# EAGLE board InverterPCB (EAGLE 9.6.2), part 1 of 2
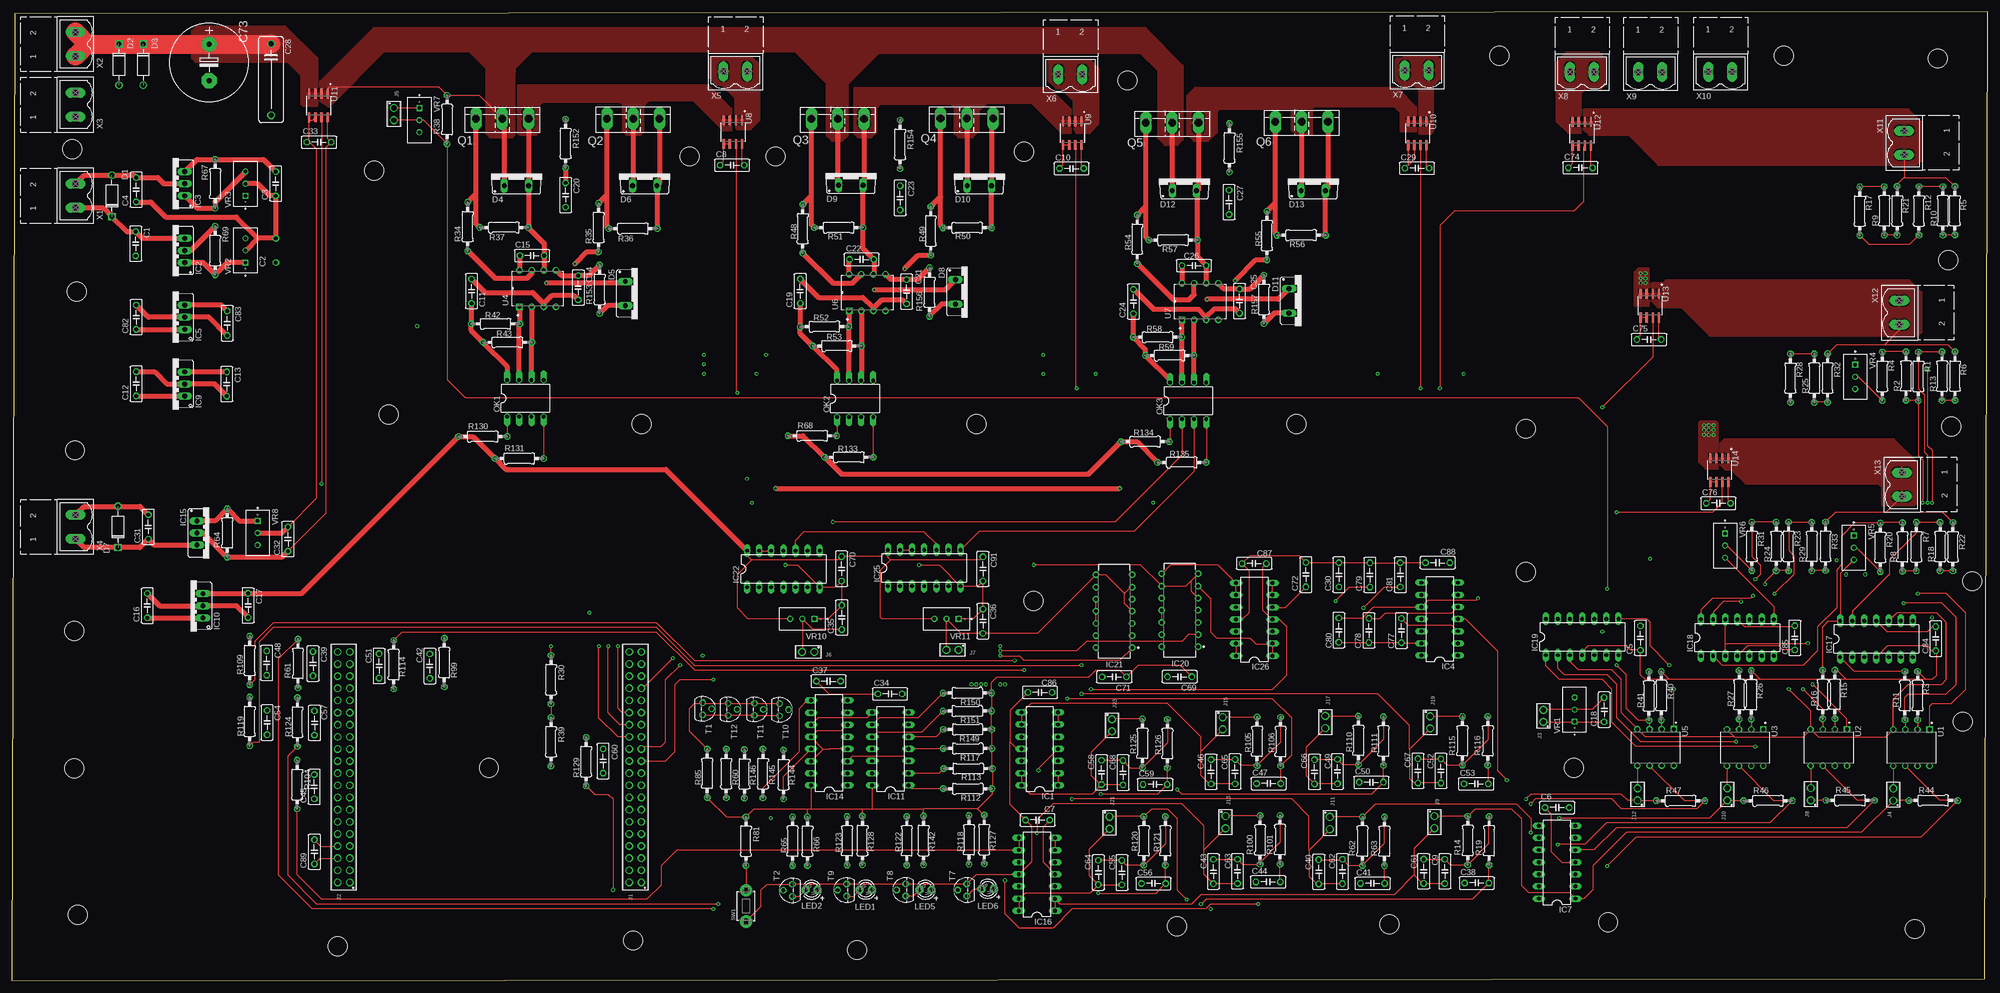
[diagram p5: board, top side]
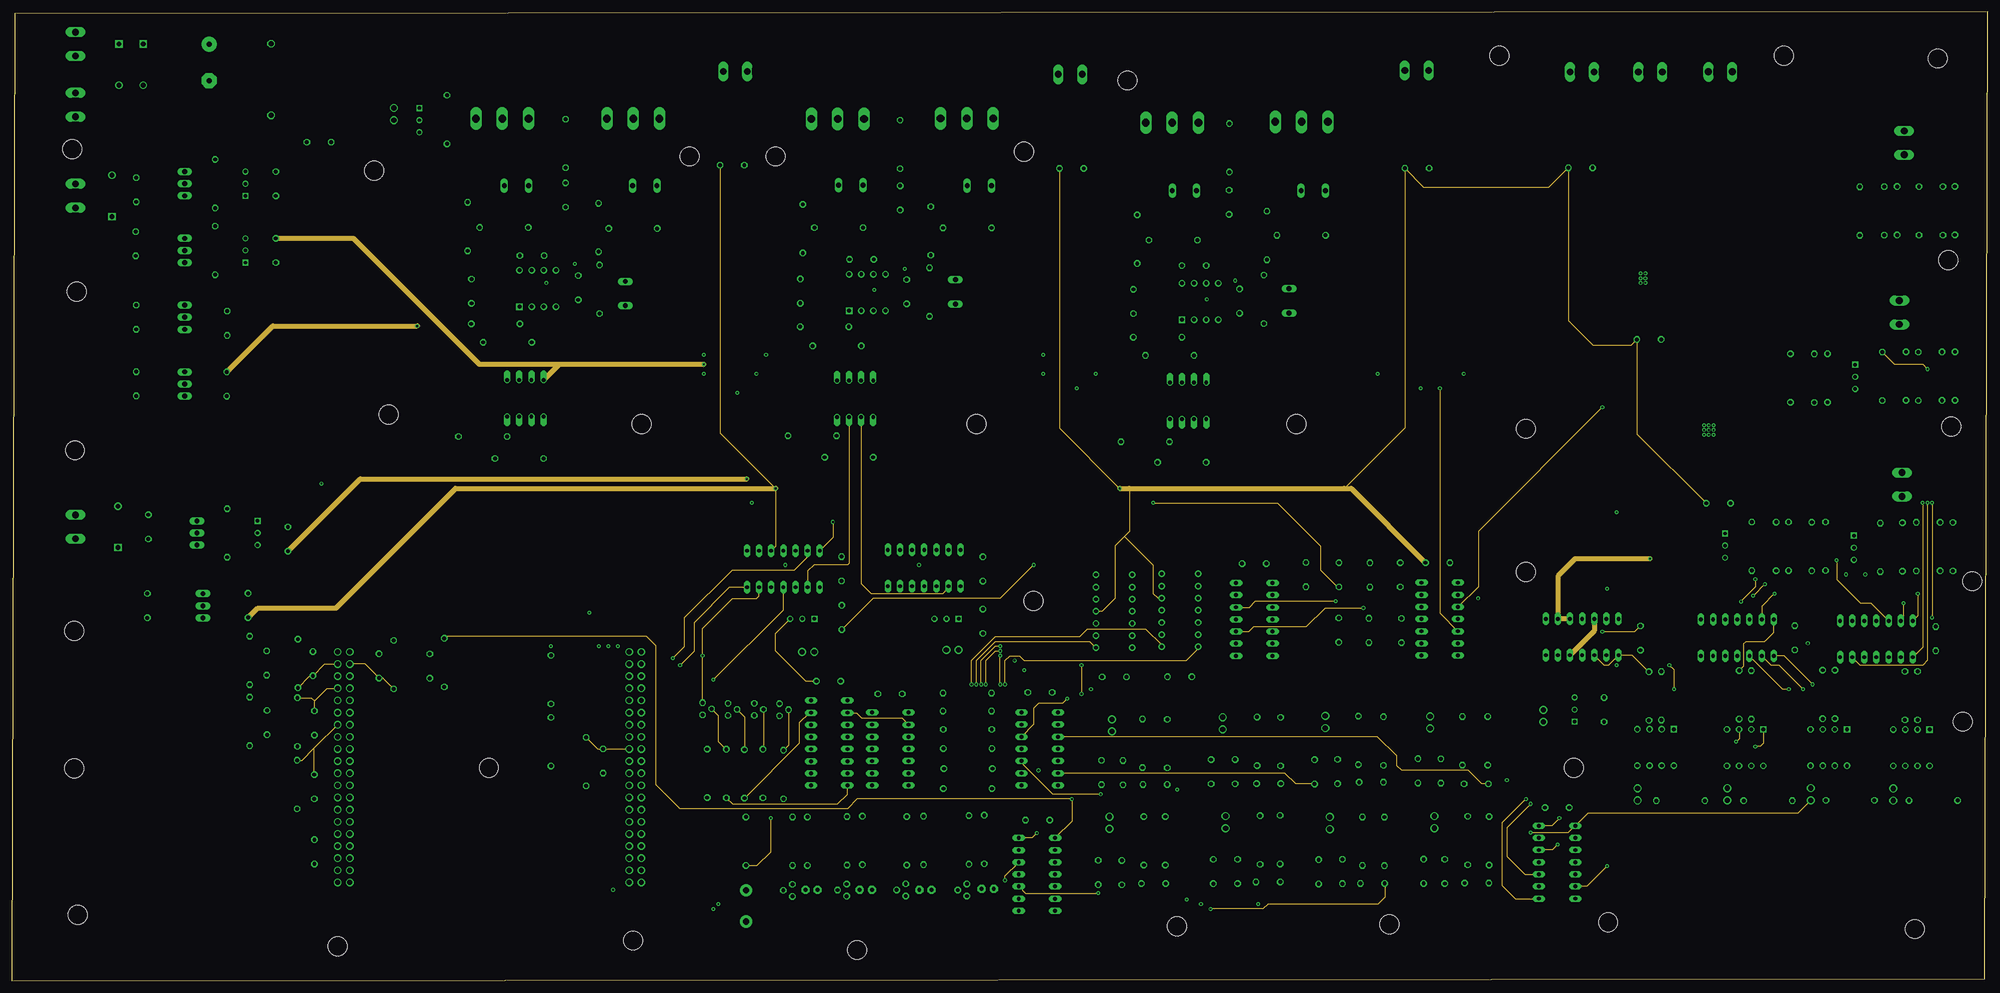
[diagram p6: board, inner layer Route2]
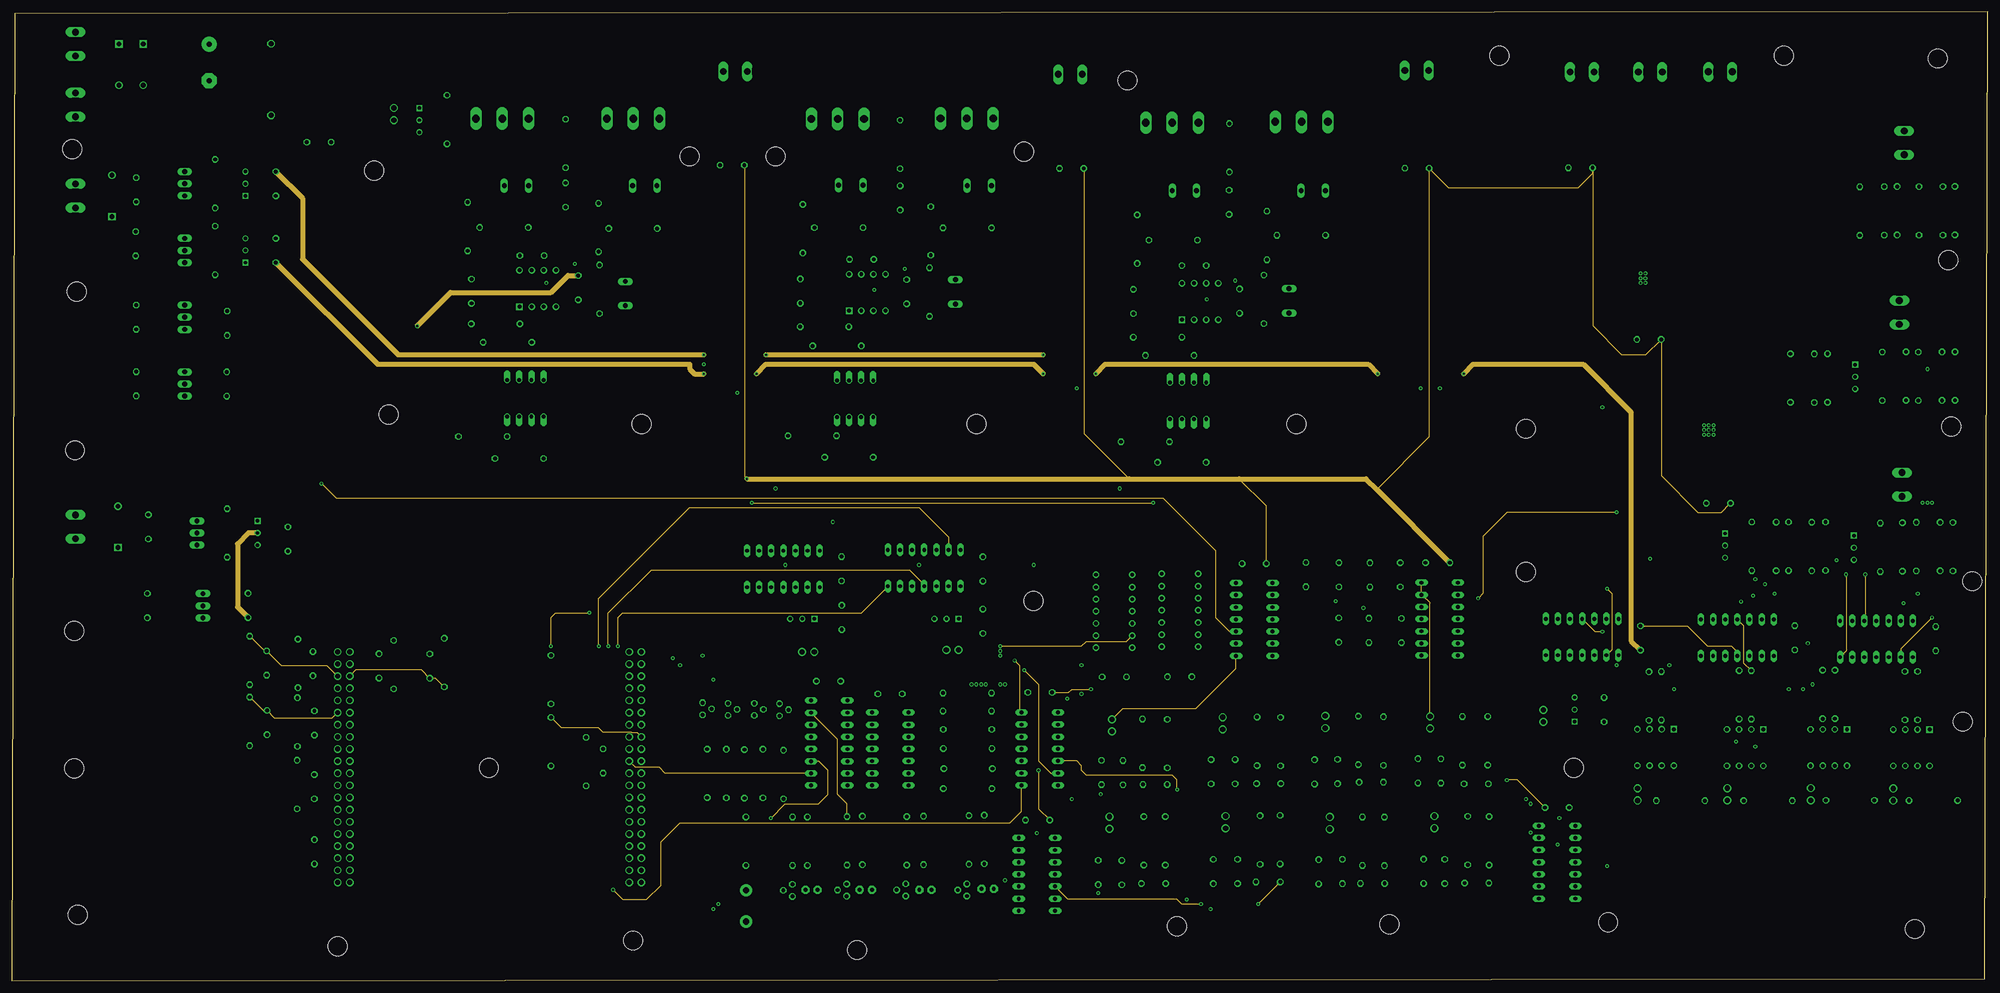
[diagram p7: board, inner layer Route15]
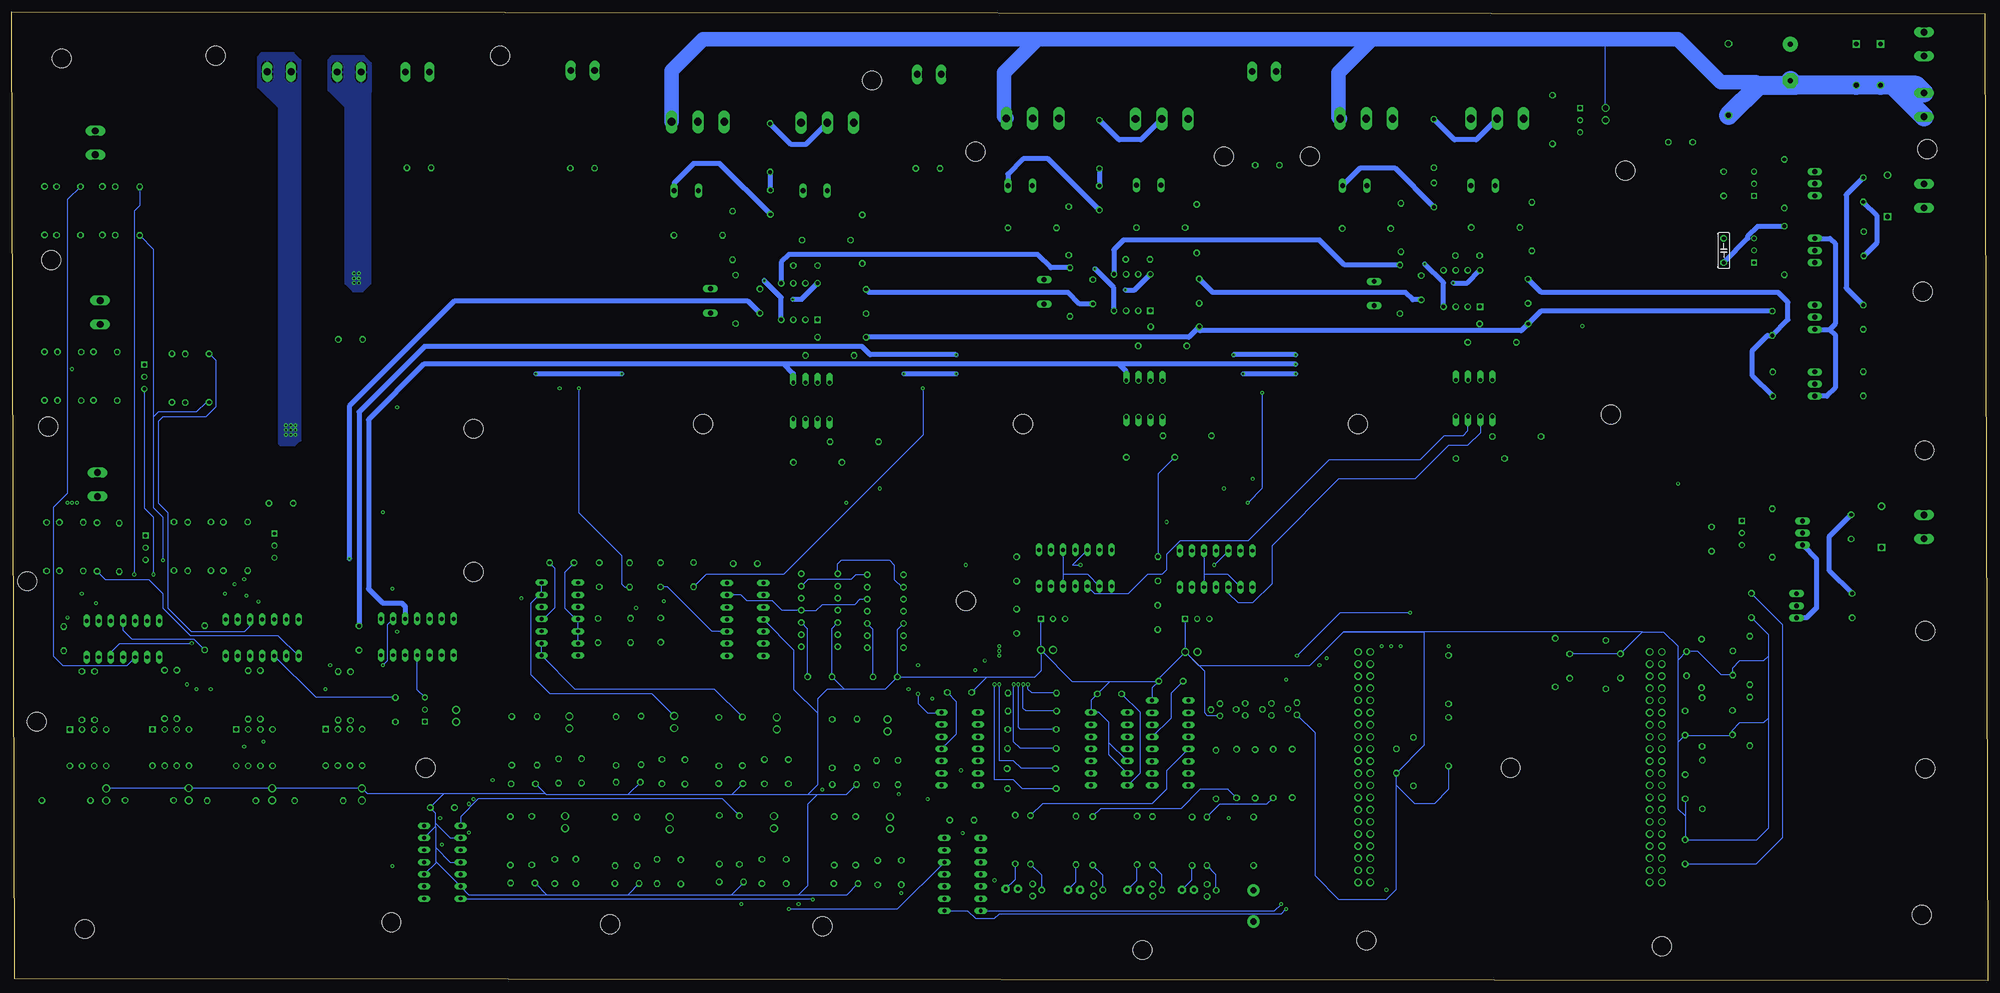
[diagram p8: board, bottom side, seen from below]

Size 413.38 x 202.75 mm. Coordinates in mm from the lower left corner, seen from the top.
Outline: 0,0 412.78,0.4 413.38,202.75 0.6,202.35 0,0
Copper layers (1+2*15+16): Top 0.07mm / dielectric 0.2mm / Route2 0.017mm / dielectric 1.465mm / Route15 0.017mm / dielectric 0.2mm / Bottom 0.07mm
Design rules "default *": minimum track width 6mil, minimum drill 0.35mm, track to track 6mil, track to pad 6mil, pad to pad 6mil, via to via 6mil, smd to smd 6mil, copper to edge 40mil, drill to drill 6mil, minimum pad ring 10mil, minimum via ring 8mil, stop-mask expansion 4mil, vias tented up to drill 0mil, thermal gap 10mil
Net classes: 1 High_gnd: clearance 1 mm
Holes 4 mm at 12.59,174.01 13.59,144.21 13.19,111.01 12.99,73.21 12.99,44.41 13.79,13.81 68.19,7.21 129.99,8.41 176.79,6.41 243.79,11.41 288.19,11.81 333.99,12.21 398.19,10.81 408.19,54.21 370.79,193.61 402.99,193.01 410.19,83.61 405.79,116.01 405.19,150.81 311.19,193.61 233.39,188.41 211.79,173.51 159.79,172.51 141.79,172.51 75.79,169.51 99.79,44.51 78.79,118.51 131.79,116.51 201.79,116.51 268.79,116.51 316.79,115.51 316.79,85.51 326.79,44.51 213.79,79.51

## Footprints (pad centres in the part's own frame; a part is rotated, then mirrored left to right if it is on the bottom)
C050-025X075 = drill 0.813 octagon: 1 -2.54,0; 2 2.54,0
C150-054X183 = drill 1.016 octagon: 1 -7.493,0; 2 7.493,0
E7,5-16 = drill 1.016 pad 3.15: + -3.81,0 | drill 1.016 pad 3.15 octagon: - 3.81,0
DO-41 = drill 1: A 4.325,0 | drill 1 square: C -4.325,0
TO220ACS = drill 1.016 long: A 2.54,-2.54; C -2.54,-2.54
DIL14 = drill 0.813 long: 1 -7.62,-3.81; 2 -5.08,-3.81; 3 -2.54,-3.81; 4 0,-3.81; 5 2.54,-3.81; 6 5.08,-3.81; 7 7.62,-3.81; 8 7.62,3.81; 9 5.08,3.81; 10 2.54,3.81; 11 0,3.81; 12 -2.54,3.81; 13 -5.08,3.81; 14 -7.62,3.81
317TS = drill 1.016 long: 1 -2.54,-2.54; 2 0,-2.54; 3 2.54,-2.54
337TS = drill 1.016 long: 1 -2.54,-2.54; 2 0,-2.54; 3 2.54,-2.54
TO220V = drill 1.016 long: 1 -2.54,-2.54; 2 0,-2.54; 3 2.54,-2.54
DIL16 = drill 0.813 long: 1 -8.89,-3.81; 2 -6.35,-3.81; 3 -3.81,-3.81; 4 -1.27,-3.81; 5 1.27,-3.81; 6 3.81,-3.81; 7 6.35,-3.81; 8 8.89,-3.81; 9 8.89,3.81; 10 6.35,3.81; 11 3.81,3.81; 12 1.27,3.81; 13 -1.27,3.81; 14 -3.81,3.81; 15 -6.35,3.81; 16 -8.89,3.81
DIP762W53P254L1969H508Q14B = drill 0.743 pad 1.343: 1 -3.81,7.62; 2 -3.81,5.08; 3 -3.81,2.54; 4 -3.81,0; 5 -3.81,-2.54; 6 -3.81,-5.08; 7 -3.81,-7.62; 8 3.81,-7.62; 9 3.81,-5.08; 10 3.81,-2.54; 11 3.81,0; 12 3.81,2.54; 13 3.81,5.08; 14 3.81,7.62
61304021821 = drill 1.02: 1 -24.13,-1.27; 2 -24.13,1.27; 3 -21.59,-1.27; 4 -21.59,1.27; 5 -19.05,-1.27; 6 -19.05,1.27; 7 -16.51,-1.27; 8 -16.51,1.27; 9 -13.97,-1.27; 10 -13.97,1.27; 11 -11.43,-1.27; 12 -11.43,1.27; 13 -8.89,-1.27; 14 -8.89,1.27; 15 -6.35,-1.27; 16 -6.35,1.27; 17 -3.81,-1.27; 18 -3.81,1.27; 19 -1.27,-1.27; 20 -1.27,1.27; 21 1.27,-1.27; 22 1.27,1.27; 23 3.81,-1.27; 24 3.81,1.27; 25 6.35,-1.27; 26 6.35,1.27; 27 8.89,-1.27; 28 8.89,1.27; 29 11.43,-1.27; 30 11.43,1.27; 31 13.97,-1.27; 32 13.97,1.27; 33 16.51,-1.27; 34 16.51,1.27; 35 19.05,-1.27; 36 19.05,1.27; 37 21.59,-1.27; 38 21.59,1.27; 39 24.13,-1.27; 40 24.13,1.27
61300211121 = drill 1.1: 1 -1.27,0; 2 1.27,0
LED3MM = drill 0.813 pad 1.676 octagon: A -1.27,0; K 1.27,0
DIL08 = drill 0.813 offset: 1 -3.81,-3.81; 2 -1.27,-3.81; 3 1.27,-3.81; 4 3.81,-3.81; 5 3.81,3.81; 6 1.27,3.81; 7 -1.27,3.81; 8 -3.81,3.81
TO-247AD-V = drill 1.6 long: D 0,-2.54; G -5.5,-2.54; S 5.5,-2.54
0207/10 = drill 0.813 octagon: 1 -5.08,0; 2 5.08,0
TACT_PANA-EVQ = drill 1.3 pad 2.54: P$1 -3.25,0; P$2 3.25,0
TO92 = drill 0.813 octagon: 1 1.27,0; 2 0,1.905; 3 -1.27,0
DIP762W52P254L1016H469Q8 = drill 0.81 square: 1 -3.81,3.81 | drill 0.81: 2 -3.81,1.27; 3 -3.81,-1.27; 4 -3.81,-3.81; 5 3.81,-3.81; 6 3.81,-1.27; 7 3.81,1.27; 8 3.81,3.81
DIP762W45P254L1092H533Q8 = drill 0.83 square: 1 -3.81,3.81 | drill 0.83: 2 -3.81,1.27; 3 -3.81,-1.27; 4 -3.81,-3.81; 5 3.81,-3.81; 6 3.81,-1.27; 7 3.81,1.27; 8 3.81,3.81
SOIC127P600X175-8N = smd 1.97 x 0.6: 1 -2.475,1.905; 2 -2.475,0.635; 3 -2.475,-0.635; 4 -2.475,-1.905; 5 2.475,-1.905; 6 2.475,-0.635; 7 2.475,0.635; 8 2.475,1.905
TRIM_3296W-1-502LF = drill 0.71 square: 1 -2.54,0 | drill 0.71: 2 0,0; 3 2.54,0
MSTBV2 = drill 1.397 long: 1 -2.5,0; 2 2.5,0

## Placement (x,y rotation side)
C1  1 µF  [C050-025X075]  25.9,154.23 270 top
C2  1 µF  [C050-025X075]  55.21,152.83 90 bottom
C3  1 µF  [C050-025X075]  55.21,166.8 90 top
C4  1 µF  [C050-025X075]  26,165.53 90 top
C5  220nF  [C050-025X075]  340.76,71.72 90 top
C6  220nF  [C050-025X075]  323.31,36.22 0 top
C7  220nF  [C050-025X075]  214.61,33.61 180 top
C8  220 nF  [C050-025X075]  150.7,170.69 0 top
C9  100 nF  [C050-025X075]  299.8,22.86 270 top
C10  220 nF  [C050-025X075]  221.72,169.99 0 top
C11  220nF  [C050-025X075]  96.16,144.31 90 top
C12  1 µF  [C050-025X075]  26,124.92 90 top
C13  220nF  [C050-025X075]  44.95,124.86 270 top
C14  1 µF  [C050-025X075]  118.5,145.04 270 top
C15  100 nF  [C050-025X075]  108.82,151.76 0 top
C16  220nF  [C050-025X075]  28.34,78.49 90 top
C17  220nF  [C050-025X075]  49.4,78.53 270 top
C18  220nF  [C050-025X075]  333.16,56.71 270 top
C19  220nF  [C050-025X075]  164.95,144.32 90 top
C20  100 nF  [C050-025X075]  115.83,164.43 270 top
C21  1 µF  [C050-025X075]  187.21,144.19 270 top
C22  100 nF  [C050-025X075]  177.79,150.96 0 top
C23  100 nF  [C050-025X075]  185.85,163.83 270 top
C24  220nF  [C050-025X075]  234.66,142.15 90 top
C25  1 µF  [C050-025X075]  256.87,142.23 270 top
C26  100 nF  [C050-025X075]  247.34,149.67 0 top
C27  100 nF  [C050-025X075]  254.67,162.92 270 top
C28  [C150-054X183]  54.21,188.6 270 top
C29  220 nF  [C050-025X075]  293.99,170.04 0 top
C30  Disp.  [C050-025X075]  277.67,84.95 90 top
C31  1 µF  [C050-025X075]  28.54,94.97 90 top
C32  220 nF  [C050-025X075]  57.75,92.43 90 top
C33  220 nF  [C050-025X075]  64.25,175.49 0 top
C34  220nF  [C050-025X075]  183.73,60.03 0 top
C35  220nF  [C050-025X075]  173.64,76.03 90 top
C36  220nF  [C050-025X075]  203.15,75.23 90 top
C37  220nF  [C050-025X075]  170.86,62.68 0 top
C38  100 nF  [C050-025X075]  306.5,20.44 0 top
C39  68 nF  [C050-025X075]  62.98,66.35 270 top
C40  100 nF  [C050-025X075]  273.43,22.78 270 top
C41  100 nF  [C050-025X075]  284.7,20.35 0 top
C42  68 nF  [C050-025X075]  87.44,65.84 270 top
C43  100 nF  [C050-025X075]  251.37,22.84 270 top
C44  100 nF  [C050-025X075]  262.84,20.66 0 top
C45  68 nF  [C050-025X075]  63.27,40.59 90 top
C46  100 nF  [C050-025X075]  250.91,43.72 270 top
C47  100 nF  [C050-025X075]  262.96,41.25 0 top
C48  68 nF  [C050-025X075]  53.31,66.48 90 top
C49  100 nF  [C050-025X075]  277.36,43.77 270 top
C50  100 nF  [C050-025X075]  284.43,41.53 0 top
C51  68 nF  [C050-025X075]  76.8,65.87 270 top
C52  100 nF  [C050-025X075]  298.99,43.9 270 top
C53  100 nF  [C050-025X075]  306.38,41.2 0 top
C54  68 nF  [C050-025X075]  53.38,54.02 90 top
C55  100 nF  [C050-025X075]  232.24,22.62 270 top
C56  100 nF  [C050-025X075]  238.87,20.34 0 top
C57  68 nF  [C050-025X075]  63.3,53.93 90 top
C58  100 nF  [C050-025X075]  227.97,43.58 270 top
C59  100 nF  [C050-025X075]  239.2,41.06 0 top
C60  68 nF  [C050-025X075]  123.7,45.97 90 top
C61  100 nF  [C050-025X075]  295.39,22.88 270 top
C62  100 nF  [C050-025X075]  278.39,22.85 270 top
C63  100 nF  [C050-025X075]  256.45,22.86 270 top
C64  100 nF  [C050-025X075]  227.31,22.64 270 top
C65  100 nF  [C050-025X075]  255.93,43.75 270 top
C66  100 nF  [C050-025X075]  272.56,43.71 270 top
C67  100 nF  [C050-025X075]  294.2,43.91 270 top
C68  100 nF  [C050-025X075]  232.47,43.54 270 top
C69  220nF  [C050-025X075]  244.34,63.61 180 top
C70  220nF  [C050-025X075]  173.59,86.21 270 top
C71  220nF  [C050-025X075]  230.65,63.56 180 top
C72  Disp.  [C050-025X075]  270.76,84.97 90 top
C73  [E7,5-16]  41.24,192.2 270 top
C74  220 nF  [C050-025X075]  328.2,170.14 0 top
C75  220 nF  [C050-025X075]  342.55,134.2 0 top
C76  220 nF  [C050-025X075]  357.06,99.92 0 top
C77  Disp.  [C050-025X075]  290.75,73.27 270 top
C78  Disp.  [C050-025X075]  283.93,73.3 270 top
C79  Disp.  [C050-025X075]  284.15,84.91 90 top
C80  Disp.  [C050-025X075]  277.62,73.36 270 top
C81  Disp.  [C050-025X075]  290.5,84.94 90 top
C82  1 µF  [C050-025X075]  26,138.86 90 top
C83  220nF  [C050-025X075]  45.05,137.59 270 top
C84  220nF  [C050-025X075]  402.53,71.58 90 top
C85  220nF  [C050-025X075]  373.06,71.76 270 top
C86  220nF  [C050-025X075]  215.11,60.34 180 top
C87  220nF  [C050-025X075]  259.93,87.3 180 top
C88  220nF  [C050-025X075]  298.33,87.47 180 top
C89  1 µF  [C050-025X075]  63.29,26.96 90 top
C91  220nF  [C050-025X075]  203.15,86.17 270 top
D1  1N4007  [DO-41]  20.92,164.26 90 top
D2  1N4007  [DO-41]  22.39,191.74 270 top
D3  1N4007  [DO-41]  27.47,191.74 270 top
D4  BYT08P  [TO220ACS]  105.57,168.92 0 top
D5  BYT08P  [TO220ACS]  130.87,143.82 270 top
D6  BYT08P  [TO220ACS]  132.41,168.94 0 top
D7  1N4007  [DO-41]  22.19,94.97 90 top
D8  BYT08P  [TO220ACS]  199.95,144.15 270 top
D9  BYT08P  [TO220ACS]  175.53,169.03 0 top
D10  BYT08P  [TO220ACS]  202.43,168.95 0 top
D11  BYT08P  [TO220ACS]  269.76,142.3 270 top
D12  BYT08P  [TO220ACS]  245.33,167.9 0 top
D13  BYT08P  [TO220ACS]  272.29,167.9 0 top
IC1  MCP604P  [DIL14]  215.06,48.51 90 top
IC2  [317TS]  33.62,152.83 90 top
IC3  [337TS]  33.62,166.8 90 top
IC4  MCP604P  [DIL14]  298.75,75.68 90 top
IC5  7805TV  [TO220V]  33.62,138.86 90 top
IC7  MCP604P  [DIL14]  323.3,24.8 90 top
IC9  7815TV  [TO220V]  33.62,124.89 90 top
IC10  7805TV  [TO220V]  37.43,78.46 90 top
IC11  74HC08N  [DIL14]  183.81,48.5 90 top
IC14  4044N  [DIL16]  171,49.74 90 top
IC15  [317TS]  41.24,93.7 270 top
IC16  MCP604P  [DIL14]  214.48,22.25 90 top
IC17  MCP604P  [DIL14]  390.13,71.51 0 top
IC18  MCP604P  [DIL14]  361.04,71.79 0 top
IC19  MCP604P  [DIL14]  328.55,71.93 0 top
IC20  LM339_PDIP  [DIP762W53P254L1969H508Q14B]  244.39,77.51 180 top
IC21  LM339_PDIP  [DIP762W53P254L1969H508Q14B]  230.64,77.31 180 top
IC22  74HC08N  [DIL14]  161.41,86.17 0 top
IC25  74HC08N  [DIL14]  190.89,86.37 0 top
IC26  MCP604P  [DIL14]  259.96,75.63 90 top
J1  [61304021821]  130.43,44.68 90 top
J2  [61304021821]  69.42,44.68 90 top
J3  [61300211121]  320.43,55.43 90 top
J4  [61300211121]  393.63,38.95 90 top
J5  [61300211121]  79.93,181.39 270 top
J6  [61300211121]  166.61,68.81 180 top
J7  [61300211121]  196.79,69.21 180 top
J8  [61300211121]  376.39,39.03 90 top
J9  [61300211121]  297.65,33.19 270 top
J10  [61300211121]  358.91,39.01 90 top
J11  [61300211121]  275.75,32.98 270 top
J12  [61300211121]  340.15,38.98 90 top
J13  [61300211121]  253.95,33.17 270 top
J15  [61300211121]  253.35,53.87 270 top
J17  [61300211121]  274.79,54.13 270 top
J19  [61300211121]  296.74,54.06 270 top
J21  [61300211121]  229.64,33.06 270 top
J23  [61300211121]  230.16,53.43 270 top
LED1  [LED3MM]  178.66,19.02 180 top
LED2  [LED3MM]  167.31,18.98 180 top
LED5  [LED3MM]  191.13,18.98 180 top
LED6  [LED3MM]  204.17,19.2 180 top
OK1  HCPL2630  [DIL08]  107.42,121.89 0 top
OK2  HCPL2630  [DIL08]  176.42,121.8 0 top
OK3  HCPL2630  [DIL08]  246.08,121.36 0 top
Q1  IRFP250  [TO-247AD-V]  102.6,182.96 0 top
Q2  IRFP250  [TO-247AD-V]  129.99,182.96 0 top
Q3  IRFP250  [TO-247AD-V]  172.79,182.93 0 top
Q4  IRFP250  [TO-247AD-V]  199.8,183 0 top
Q5  IRFP250  [TO-247AD-V]  242.75,182.11 0 top
Q6  IRFP250  [TO-247AD-V]  269.84,182.31 0 top
R1  100 kOhm  [0207/10]  398.9,126.48 270 top
R2  10 kOhm  [0207/10]  396.32,126.54 90 top
R3  33 Ohm  [0207/10]  398.75,59.65 90 top
R4  7.5 kOhm  [0207/10]  391.34,126.5 270 top
R5  1.2MOhm  [0207/10]  406.54,161.16 270 top
R6  1.2MOhm  [0207/10]  406.56,126.54 270 top
R7  100 kOhm  [0207/10]  398.46,90.84 270 top
R8  10 kOhm  [0207/10]  395.57,90.77 90 top
R9  1.2MOhm  [0207/10]  391.78,161.12 90 top
R10  1.2MOhm  [0207/10]  404.03,161.12 90 top
R11  13 kOhm  [0207/10]  396.09,59.65 90 top
R12  100 kOhm  [0207/10]  399.03,161.12 270 top
R13  1.2MOhm  [0207/10]  403.86,126.52 90 top
R14  220 Ohm  [0207/10]  304.61,29.33 90 top
R15  33 Ohm  [0207/10]  381.45,59.92 90 top
R16  13 kOhm  [0207/10]  378.87,59.9 90 top
R17  100 kOhm  [0207/10]  386.63,161.07 270 top
R18  1.2MOhm  [0207/10]  403.46,90.85 90 top
R19  220 Ohm  [0207/10]  309.08,29.27 90 top
R20  7.5 kOhm  [0207/10]  390.95,90.69 270 top
R21  1.2MOhm  [0207/10]  394.46,161.14 270 top
R22  1.2MOhm  [0207/10]  406.14,90.83 270 top
R23  100 kOhm  [0207/10]  371.73,90.91 270 top
R24  10 kOhm  [0207/10]  369.15,90.89 90 top
R25  1.2MOhm  [0207/10]  377.14,126.09 90 top
R26  33 Ohm  [0207/10]  363.94,59.81 90 top
R27  13 kOhm  [0207/10]  361.41,59.83 90 top
R28  100 kOhm  [0207/10]  372.13,126.12 270 top
R29  1.2MOhm  [0207/10]  376.59,90.86 90 top
R30  220 Ohm  [0207/10]  112.79,63.01 270 top
R31  7.5 kOhm  [0207/10]  364.06,90.9 270 top
R32  1.2MOhm  [0207/10]  379.9,126.14 270 top
R33  1.2MOhm  [0207/10]  379.48,90.92 270 top
R34  6.8 Ohm  [0207/10]  95.34,157.83 270 top
R35  6.8 Ohm  [0207/10]  122.74,157.63 270 top
R36  47kOhm  [0207/10]  129.95,157.42 0 top
R37  47kOhm  [0207/10]  102.96,157.63 0 top
R38  10 kOhm  [0207/10]  91.04,180.23 90 top
R39  220 Ohm  [0207/10]  112.79,50.01 270 top
R40  33 Ohm  [0207/10]  345.12,59.62 90 top
R41  13 kOhm  [0207/10]  342.53,59.57 90 top
R42  3.9 kOhm  [0207/10]  101.2,137.48 0 top
R43  3.9 kOhm  [0207/10]  103.69,133.6 0 top
R44  13 kOhm  [0207/10]  402.03,37.71 0 top
R45  13 kOhm  [0207/10]  384.64,37.76 0 top
R46  13 kOhm  [0207/10]  367.43,37.66 0 top
R47  13 kOhm  [0207/10]  349.16,37.66 0 top
R48  6.8 Ohm  [0207/10]  165.47,157.38 270 top
R49  6.8 Ohm  [0207/10]  192.25,156.93 270 top
R50  47kOhm  [0207/10]  199.9,157.56 0 top
R51  47kOhm  [0207/10]  172.99,157.61 0 top
R52  3.9 kOhm  [0207/10]  170.02,136.87 0 top
R53  3.9 kOhm  [0207/10]  172.63,132.84 0 top
R54  6.8 Ohm  [0207/10]  235.45,155.19 270 top
R55  6.8 Ohm  [0207/10]  262.59,155.96 270 top
R56  47kOhm  [0207/10]  269.78,156 0 top
R57  47kOhm  [0207/10]  242.98,155 0 top
R58  3.9 kOhm  [0207/10]  239.72,134.66 0 top
R59  3.9 kOhm  [0207/10]  242.26,130.86 0 top
R60  39 kOhm  [0207/10]  149.47,43.36 270 top
R61  470 Ohm  [0207/10]  59.84,66.39 90 top
R62  220 Ohm  [0207/10]  282.58,29.19 90 top
R63  220 Ohm  [0207/10]  287.18,29.15 90 top
R64  2.5 kOhm  [0207/10]  45.05,93.7 90 top
R65  39 kOhm  [0207/10]  163.34,29.19 90 top
R66  150 Ohm  [0207/10]  166.44,29.19 270 top
R67  2.5 kOhm  [0207/10]  42.51,166.8 90 top
R68  220 Ohm  [0207/10]  167.46,114.04 0 top
R69  2.5 kOhm  [0207/10]  42.51,152.83 270 top
R81  100 kOhm  [0207/10]  153.57,29.19 270 top
R85  100 kOhm  [0207/10]  145.47,43.39 90 top
R99  470 Ohm  [0207/10]  90.45,66.57 90 top
R100  220 Ohm  [0207/10]  261.17,29.44 90 top
R101  220 Ohm  [0207/10]  265.34,29.5 90 top
R104  470 Ohm  [0207/10]  59.66,41.06 270 top
R105  220 Ohm  [0207/10]  260.54,50.09 90 top
R106  220 Ohm  [0207/10]  265.46,50.04 90 top
R109  470 Ohm  [0207/10]  49.75,67.03 270 top
R110  220 Ohm  [0207/10]  281.72,50.29 90 top
R111  220 Ohm  [0207/10]  286.98,50.15 90 top
R112  100 kOhm  [0207/10]  199.97,40.19 180 top
R113  100 kOhm  [0207/10]  200.07,44.39 180 top
R114  470 Ohm  [0207/10]  79.88,66.14 90 top
R115  220 Ohm  [0207/10]  303.49,50.2 90 top
R116  220 Ohm  [0207/10]  308.79,50.2 90 top
R117  100 kOhm  [0207/10]  199.97,48.59 180 top
R118  39 kOhm  [0207/10]  200.24,29.47 90 top
R119  470 Ohm  [0207/10]  49.74,54.26 270 top
R120  220 Ohm  [0207/10]  236.84,29.27 90 top
R121  220 Ohm  [0207/10]  241.34,29.27 90 top
R122  39 kOhm  [0207/10]  187.24,29.27 90 top
R123  39 kOhm  [0207/10]  174.74,29.27 90 top
R124  470 Ohm  [0207/10]  59.74,54.13 270 top
R125  220 Ohm  [0207/10]  236.54,49.67 90 top
R126  220 Ohm  [0207/10]  241.74,49.61 90 top
R127  150 Ohm  [0207/10]  203.44,29.55 270 top
R128  150 Ohm  [0207/10]  177.94,29.35 270 top
R129  470 Ohm  [0207/10]  120.13,45.85 270 top
R130  220 Ohm  [0207/10]  98.52,113.88 0 top
R131  220 Ohm  [0207/10]  106.15,109.29 0 top
R133  220 Ohm  [0207/10]  175.13,109.55 0 top
R134  220 Ohm  [0207/10]  237.13,112.8 0 top
R135  220 Ohm  [0207/10]  244.79,108.47 0 top
R142  150 Ohm  [0207/10]  190.74,29.35 270 top
R144  39 kOhm  [0207/10]  161.44,43.15 270 top
R145  39 kOhm  [0207/10]  157.14,43.35 270 top
R146  39 kOhm  [0207/10]  153.27,43.28 270 top
R149  100 kOhm  [0207/10]  199.94,52.59 180 top
R150  100 kOhm  [0207/10]  199.89,60.21 180 top
R151  100 kOhm  [0207/10]  199.88,56.44 180 top
R152  10 Ohm  [0207/10]  115.84,175.23 270 top
R153  1.8 Ohm  [0207/10]  122.95,144.7 270 top
R154  10 Ohm  [0207/10]  185.84,175.03 270 top
R155  10 Ohm  [0207/10]  254.73,174.32 270 top
R156  1.8 Ohm  [0207/10]  192,144.12 270 top
R157  1.8 Ohm  [0207/10]  261.95,142.61 270 top
SW1  [TACT_PANA-EVQ]  153.59,15.64 90 top
T1  BC547  [TO92]  144.5,56.9 270 top
T2  BC547  [TO92]  163.31,18.9 90 top
T7  BC547  [TO92]  199.81,18.97 90 top
T8  BC547  [TO92]  187.03,18.99 90 top
T9  BC547  [TO92]  174.66,18.96 90 top
T10  BC547  [TO92]  160.6,56.7 270 top
T11  BC547  [TO92]  155.33,56.78 270 top
T12  BC547  [TO92]  149.83,56.78 270 top
U1  IL300  [DIP762W52P254L1016H469Q8]  397.45,48.75 270 top
U2  IL300  [DIP762W52P254L1016H469Q8]  380.16,48.8 270 top
U3  IL300  [DIP762W52P254L1016H469Q8]  362.66,48.79 270 top
U4  IR2183  [DIP762W45P254L1092H533Q8]  110.02,144.87 90 top
U5  IL300  [DIP762W52P254L1016H469Q8]  343.92,48.81 270 top
U6  IR2183  [DIP762W45P254L1092H533Q8]  178.99,144.03 90 top
U7  IR2183  [DIP762W45P254L1092H533Q8]  248.62,142.15 90 top
U8  ACS722LLCTR-05AB-T  [SOIC127P600X175-8N]  150.85,177.58 270 top
U9  ACS722LLCTR-05AB-T  [SOIC127P600X175-8N]  221.86,177.38 270 top
U10  ACS722LLCTR-05AB-T  [SOIC127P600X175-8N]  294.05,177.34 270 top
U11  ACS722LLCTR-05AB-T  [SOIC127P600X175-8N]  64.13,183.17 270 top
U12  ACS722LLCTR-05AB-T  [SOIC127P600X175-8N]  328.45,177.24 270 top
U13  ACS722LLCTR-05AB-T  [SOIC127P600X175-8N]  342.68,141.27 270 top
U14  ACS722LLCTR-05AB-T  [SOIC127P600X175-8N]  357.25,106.84 270 top
VR1  0 - 5 kOhm  [TRIM_3296W-1-502LF]  326.97,56.74 90 top
VR2  0 - 5 kOhm  [TRIM_3296W-1-502LF]  48.86,152.83 90 top
VR3  0 - 5 kOhm  [TRIM_3296W-1-502LF]  48.86,166.8 90 top
VR4  0 - 5 kOhm  [TRIM_3296W-1-502LF]  385.69,126.39 270 top
VR5  0 - 5 kOhm  [TRIM_3296W-1-502LF]  385.4,90.62 270 top
VR6  0 - 5 kOhm  [TRIM_3296W-1-502LF]  358.46,91.05 270 top
VR7  0 - 5 kOhm  [TRIM_3296W-1-502LF]  85.26,180.09 270 top
VR8  0 - 5 kOhm  [TRIM_3296W-1-502LF]  51.4,93.7 270 top
VR10  0 - 5 kOhm  [TRIM_3296W-1-502LF]  165.38,75.73 180 top
VR11  0 - 5 kOhm  [TRIM_3296W-1-502LF]  195.55,75.73 180 top
X1  [MSTBV2]  13.3,164.26 90 top
X2  [MSTBV2]  13.3,196.01 90 top
X3  [MSTBV2]  13.3,183.31 90 top
X4  [MSTBV2]  13.3,94.97 90 top
X5  [MSTBV2]  151.36,190.31 0 top
X6  [MSTBV2]  221.46,189.71 0 top
X7  [MSTBV2]  293.96,190.51 0 top
X8  [MSTBV2]  328.53,190.19 0 top
X9  [MSTBV2]  342.82,190.16 0 top
X10  [MSTBV2]  357.47,190.23 0 top
X11  [MSTBV2]  395.94,175.36 270 top
X12  [MSTBV2]  394.92,139.84 270 top
X13  [MSTBV2]  395.47,103.85 270 top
